| Texas Instruments Incorporated
| Low-Noise Clock Jitter Cleaner with Dual Loop PLLs
| Marketing part#   Voltage Range   Package-type   #pins/pkg drawing
| LMK04828   3.0V - 3.6V   LLP   64-pin SQ
[IBIS Ver]   4.1
[File name]   lmk04828.ibs
[File Rev]   1.5
[Date]   2/08/2017
[Source]   Model built from spectre simulations at:
   Texas Instruments Incorporated.
   Analog-eLab, HPA
   12500 TI Blvd
   Dallas, TX -75243
   For Support e-mail: elab_ibis@list.ti.com
[Notes]   Revision History
   Rev 1.5: 02/08/2017
   - Fix strong corner LVPECL_2p0 and LVPECL simulation problems. Time offset removed
   - Update OSCin buffer model
   - Add XTAL on and XTAL off C_comp values
   This file was modified on 2/2/2017 13:44 by the Mentor Graphics
   IBISVTC program, to remove initial non-switching delay(s) from one
   or more models V-t tables. Modified models:
   SDIO,
   LVCMOS_OSC,
   LVDS_OSC,
   LVPECL1P6_OSC,
   LVPECL2P0_OSC,
   LVDS,
   HSDS_6mA,
   HSDS_8mA,
   HSDS_10mA,
   LVPECL1P6,
   LVPECL2P0,
   LCPECL
   Original V-t tables have been left in the affected models, but commented out.
   Rev 1.4: 10/24/2016
   - Correct pin name and Diff pin statement
   Rev 1.3: 12/08/2014
   - Update package pin parasitics
   Rev 1.2: 04/24/2014
   - Correct LCPECL model name
   Rev 1.1: 10/15/2013
   - Add SYNC pin. Assign RESET to SDIO buffer
   Rev 1.0: 01/09/2013
   -Pulldown non-monotonic for LVDS_OSC model
   -Pulldown & pullup non-monotonic for LVPECL_OSC models
   -Pulldown & pullup non-monotonic for SDIO models
   -LVPECL simulation recommendation:
   It is recommended that a small (1nF or less) AC coupling cap
   be used. Larger values will result in long settling times
   - ccomp values are based on PVT settings:
   MIN: Low Voltage, High Temperature, Weak Process
   TYP: Nominal Voltage, Nominal Temperature, Nominal Process
   MAX: High Voltage, Low Temperature, Fast Process
   - C_comp although listed in numerical order of value are obtained from varying PVT conditions.
   For PVT conditions for each specific value, refer to the buffer description under respective [Model].
   IBIS model user is responsible for using appropriate C_comp to simulate for Signal Integrity.
[Disclaimer]  This model is designed as an aid for customers of Texas Instruments
 TI and its licensors and suppliers make no warranties, either expressed
 or implied, with respect to this  model, including the warranties of
 merchantability or fitness for a particular purpose.
 The model is provided solely on an "as is" basis. The entire risk as to
 its quality and performance is with the customer.
[Copyright] (C)Copyright 2017 Texas Instruments Incorporated.
   All rights reserved.
[Component]   LMK04828BISQ
[Manufacturer]  Texas Instruments Incorporated
[Package]   |64-pin LLP SQ package
|   typ   min   max
R_pkg   0.8083   0.2082   1.1685
L_pkg   1.9144n   0.9780n   2.5932n
C_pkg   0.2940p   0.2235p   0.3750p
[Pin]   signal_name   model_name   R_pin   L_pin   C_pin
1   DCLKOUT0   TRI_MODE_OUT   1.0479   2.2614n   0.3102p
2   DCLKOUT0*   TRI_MODE_OUT   0.9280   2.0696n   0.2990p
3   SDCLKOUT1   TRI_MODE_OUT   0.9076   1.9169n   0.2964p
4   SDCLKOUT1*   TRI_MODE_OUT   0.7860   1.7984n   0.2662p
5   RESET   SDIO   0.7397   1.6454n   0.2566p
6   SYNC   SYNC   0.6580   1.6443n   0.2235p
7   NC   NC   0.8083   1.9144n   0.2940p
8   NC   NC   0.2082   0.9780n   0.3750p
9   NC   NC   0.8083   1.9144n   0.2940p
10   VCC1   POWER   0.6675   1.4601n   0.2362p
11   LDOBYP1   NC   0.6633   1.6138n   0.2394p
12   LDOBYP2   NC   0.7420   1.6705n   0.2565p
13   SDCLKOUT3   TRI_MODE_OUT   0.7864   1.7943n   0.2681p
14   SDCLKOUT3*   TRI_MODE_OUT   0.9061   1.9343n   0.2945p
15   DLKOUT2   TRI_MODE_OUT   0.9417   2.0541n   0.3033p
16   DLKOUT2*   TRI_MODE_OUT   1.0450   2.2863n   0.3073p
17   VCC2   POWER   0.5439   1.9925n   0.3083p
18   CS*   SCK   0.6208   1.8410n   0.3548p
19   SCK   SCK   1.0434   2.1334n   0.3225p
20   SDIO   SDIO   0.9542   2.0383n   0.3001p
21   VCC3   POWER   0.9298   1.9770n   0.2928p
22   SDCLKOUT5   TRI_MODE_OUT   0.8633   1.9431n   0.2749p
23   SDCLKOUT5*   TRI_MODE_OUT   0.4944   1.5389n   0.3209p
24   DLKOUT4   TRI_MODE_OUT   0.4513   1.5949n   0.3085p
25   DLKOUT4*   TRI_MODE_OUT   0.7761   2.0010n   0.2589p
26   VCC4   POWER   0.7888   2.0399n   0.2595p
27   DLKOUT6   TRI_MODE_OUT   0.8372   2.0300n   0.2601p
28   DLKOUT6*   TRI_MODE_OUT   0.8778   1.9970n   0.2766p
29   SDCLKOUT7   TRI_MODE_OUT   0.9549   2.0555n   0.2956p
30   SDCLKOUT7*   TRI_MODE_OUT   0.6176   1.6773n   0.3714p
31   STATUS   SDIO   0.9873   2.2321n   0.3058p
32   CPOUT1   NC   1.0155   2.5932n   0.2924p
33   VCC5   POWER   1.0562   2.4339n   0.2970p
34   CLKIN1   CLKIN   1.0279   2.1272n   0.3171p
35   CLKIN1*   CLKIN   0.5777   1.6206n   0.3720p
36   VCC6   POWER   0.9257   2.0512n   0.2910p
37   CLKIN0   CLKIN   0.8488   1.9597n   0.2725p
38   CLKIN0*   CLKIN   0.5091   1.4436n   0.3284p
39   VCC7   POWER   0.7887   1.7936n   0.2637p
40   OSCOUT   OSCOUT   0.7794   1.6957n   0.2636p
41   OSCOUT*   OSCOUT   0.4498   1.2960n   0.3176p
42   VCC8   POWER   0.7591   1.7186n   0.2560p
43   OSCIN   OSCIN   0.7654   1.7601n   0.2533p
44   OSCIN*   OSCIN   0.7788   1.8176n   0.2606p
45   VCC9   POWER   0.8019   2.0498n   0.2623p
46   CPOUT2   NC   0.8551   2.1817n   0.2776p
47   VCC10   POWER   0.5509   1.8732n   0.3295p
48   STATUS_LD2   SDIO   1.1185   2.3922n   0.3166p
49   SDCLKOUT9   TRI_MODE_OUT   1.1228   2.4432n   0.3171p
50   SDCLKOUT9*   TRI_MODE_OUT   1.1685   2.3406n   0.3461p
51   DCLKOUT8   TRI_MODE_OUT   1.0374   2.2717n   0.3156p
52   DCLKOUT8*   TRI_MODE_OUT   0.6154   1.6880n   0.3737p
53   VCC11   POWER   0.9641   2.0390n   0.2986p
54   DCLKOUT10   TRI_MODE_OUT   0.8853   1.9486n   0.2812p
55   DCLKOUT10*   TRI_MODE_OUT   0.8702   1.8830n   0.2797p
56   SDCLKOUT11   TRI_MODE_OUT   0.8238   1.8596n   0.2666p
57   SDCLKOUT11*   TRI_MODE_OUT   0.4907   1.4278n   0.3203p
58   CLKN_SEL0   NC   0.8223   1.8286n   0.2691p
59   CLKN_SEL1   NC   0.8277   1.8868n   0.2674p
60   SDCLKOUT13   TRI_MODE_OUT   0.8684   1.8586n   0.2799p
61   SDCLKOUT13*   TRI_MODE_OUT   0.9011   2.0080n   0.2815p
62   DCLKOUT12   TRI_MODE_OUT   0.9334   2.1446n   0.2820p
63   DCLKOUT12*   TRI_MODE_OUT   0.8912   2.3255n   0.2704p
64   VCC12   POWER   0.5148   1.7149n   0.3615p
65   DAP   GND   0.0135   0.0533n   11.945p
[Package Model] llp64_lmk04828nsa2
[Diff pin]  inv_pin  vdiff  tdelay_typ  tdelay_min  tdelay_max
 1   2   0.0   0.0s   0.0s   0.0s
 3   4   0.0   0.0s   0.0s   0.0s
13   14   0.0   0.0s   0.0s   0.0s
15   16   0.0   0.0s   0.0s   0.0s
22   23   0.0   0.0s   0.0s   0.0s
24   25   0.0   0.0s   0.0s   0.0s
27   28   0.0   0.0s   0.0s   0.0s
29   30   0.0   0.0s   0.0s   0.0s
34   35   0.0   0.0s   0.0s   0.0s
37   38   0.0   0.0s   0.0s   0.0s
40   41   0.0   0.0s   0.0s   0.0s
43   44   0.0   0.0s   0.0s   0.0s
49   50   0.0   0.0s   0.0s   0.0s
51   52   0.0   0.0s   0.0s   0.0s
54   55   0.0   0.0s   0.0s   0.0s
56   57   0.0   0.0s   0.0s   0.0s
60   61   0.0   0.0s   0.0s   0.0s
62   63   0.0   0.0s   0.0s   0.0s
[Model Selector] TRI_MODE_OUT
LVDS   LVDS OUTPUT
HSDS_6mA   HSDS 6mA OUTPUT
HSDS_8mA   HSDS 8mA OUTPUT
HSDS_10mA   HSDS 10mA OUTPUT
LVPECL1P6   LVPECL 1.6V OUTPUT
LVPECL2P0   LVPECL 2.0V OUTPUT
LCPECL   LCPECL
[Model Selector] OSCOUT
LVPECL1P6_OSC   LVPECL 1.6V OUTPUT
LVPECL2P0_OSC   LVPECL 2.0V OUTPUT
LVDS_OSC   LVDS OUTPUT
LVCMOS_OSC   LVCMOS OUTPUT
[Define Package Model]  llp64_lmk04828nsa2
[Manufacturer]  Unknown
[OEM]  Unknown
[Description]  Package Model,10GHz using buildsheet AD#LMK04828NSA2-01 RevA
[Number Of Pins]  65
[Pin Numbers]
|Pin Num   Terminal Name
1   | L1:1
2   | L2:2
3   | L3:3
4   | L4:4
5   | L5:5
6   | L6:6
7   | L7:7
8   | L8:8
9   | L9:9
10   | L10:10
11   | L11:11
12   | L12:12
13   | L13:13
14   | L14:14
15   | L15:15
16   | L16:16
17   | L17:17
18   | L18:18
19   | L19:19
20   | L20:20
21   | L21:21
22   | L22:22
23   | L23:23
24   | L24:24
25   | L25:25
26   | L26:26
27   | L27:27
28   | L28:28
29   | L29:29
30   | L30:30
31   | L31:31
32   | L32:32
33   | L33:33
34   | L34:34
35   | L35:35
36   | L36:36
37   | L37:37
38   | L38:38
39   | L39:39
40   | L40:40
41   | L41:41
42   | L42:42
43   | L43:43
44   | L44:44
45   | L45:45
46   | L46:46
47   | L47:47
48   | L48:48
49   | L49:49
50   | L50:50
51   | L51:51
52   | L52:52
53   | L53:53
54   | L54:54
55   | L55:55
56   | L56:56
57   | L57:57
58   | L58:58
59   | L59:59
60   | L60:60
61   | L61:61
62   | L62:62
63   | L63:63
64   | L64:64
65   | LDAP:65
[Model Data]
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[End Model Data]
[End Package Model]
| Models and submodels in the file (16): SCK (Input), SYNC (Input), SDIO (I/O), CLKIN (Input), OSCIN (Input), LVCMOS_OSC (Output), LVDS_OSC (Output), LVPECL1P6_OSC (Output), LVPECL2P0_OSC (Output), LVDS (Output), HSDS_6mA (Output), HSDS_8mA (Output), HSDS_10mA (Output), LVPECL2P0 (Output), LVPECL1P6 (Output), LCPECL (Output)
